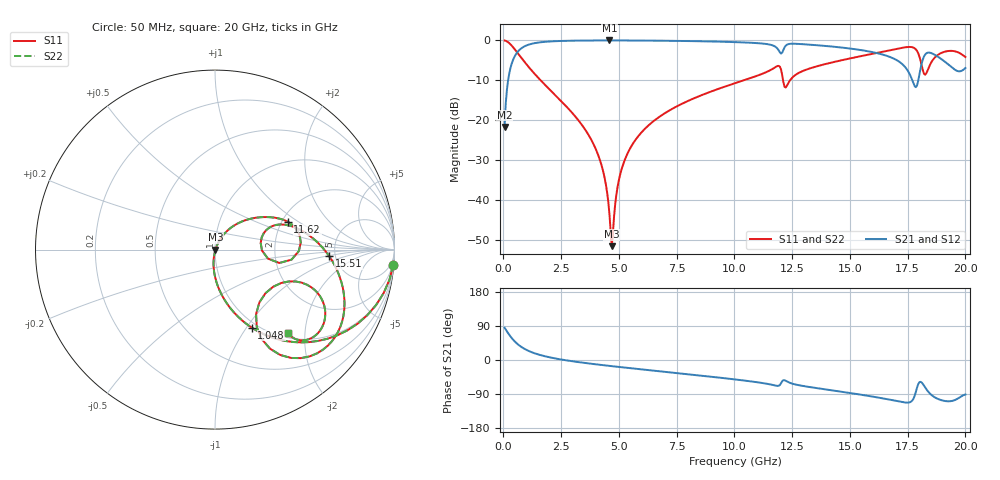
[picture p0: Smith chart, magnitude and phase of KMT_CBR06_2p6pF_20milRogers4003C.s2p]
! Data measured by Modelithics Inc. support@modelithics.com 813-866-6335
! KEMET CBR0603 2.6pF, Pad Width= 0.851mm, Pad Length= 0.64mm, Pad Gap= 0.62mm, 20mil Rogers 4003C substrate Data, January 2022
# hz S ma R 50
! 2 Port Network Data from SP1.SP block
! freq  magS11  angS11  magS21  angS21  magS12  angS12  magS22  angS22
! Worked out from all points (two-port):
!   401 points, 50 MHz to 20 GHz, reference 50 ohm
!   highest |S21| = -0.02 dB at 4.589 GHz (marker M1); lowest = -21.7 dB at 50 MHz (marker M2)
!   |S21| within 3 dB of the highest: 594.2 MHz to 11.97 GHz (11.38 GHz wide, 181 % of centre); 12.07 GHz to 16.04 GHz (3.97 GHz wide, 28.2 % of centre)
!   lowest |S11| = -51.5 dB at 4.688 GHz (marker M3), VSWR 1.01, Z = 50.2 - j0.0955 ohm
!   |S11| at or under -10 dB: 1.61 GHz to 10.4 GHz (8.794 GHz wide, 146 % of centre); 12.11 GHz to 12.41 GHz (302.9 MHz wide, 2.47 % of centre)
!   |S22| runs from -51.5 to 0.0 dB; largest |S21 - S12| = 0
!   S11 on the Smith chart (normalised r, x): 50 MHz: 1, -23; 1.048 GHz: 0.94, -1.06; 11.62 GHz: 2.15, +0.82; 15.51 GHz: 4.45, -0.56; 20 GHz: 1.09, -1.64
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5e7  0.9966 -4.9  0.08253 85.1  0.08253 85.1  0.9966 -4.9
3.99125e8  0.8321 -35.0  0.5537 54.9  0.5537 54.9  0.8321 -35.0
1.0475e9  0.4812 -64.7  0.8753 25.1  0.8753 25.1  0.4812 -64.7
3.391625e9  0.08784 -95.3  0.9938 -6.7  0.9938 -6.7  0.08784 -95.3
4.2395e9  0.02781 -97.9  0.997 -13.1  0.997 -13.1  0.02781 -97.9
4.588625e9  0.006676 -82.5  0.9972 -15.6  0.9972 -15.6  0.006676 -82.5
4.688375e9  0.002656 -21.0  0.9972 -16.2  0.9972 -16.2  0.002656 -21.0
4.987625e9  0.01726 62.6  0.9969 -18.2  0.9969 -18.2  0.01726 62.6
5.33675e9  0.03652 65.0  0.9963 -20.6  0.9963 -20.6  0.03652 65.0
6.73325e9  0.1095 58.7  0.9904 -29.5  0.9904 -29.5  0.1095 58.7
1.0025e10  0.2909 37.7  0.951 -51.2  0.951 -51.2  0.2909 37.7
1.1621e10  0.4341 20.9  0.8721 -65.3  0.8721 -65.3  0.4341 20.9
1.192025e10  0.4797 4.9  0.7465 -67.9  0.7465 -67.9  0.4797 4.9
1.22195e10  0.2572 8.3  0.8566 -54.8  0.8566 -54.8  0.2572 8.3
1.336662e10  0.455 16.2  0.8785 -72.4  0.8785 -72.4  0.455 16.2
1.551125e10  0.6376 -3.3  0.7533 -91.9  0.7533 -91.9  0.6376 -3.3
1.670825e10  0.7491 -17.5  0.6236 -104.5  0.6236 -104.5  0.7491 -17.5
1.78055e10  0.7948 -48.5  0.267 -94.3  0.267 -94.3  0.7948 -48.5
1.815462e10  0.4263 -57.5  0.5742 -62.9  0.5742 -62.9  0.4263 -57.5
1.8404e10  0.4486 -23.3  0.7033 -84.6  0.7033 -84.6  0.4486 -23.3
1.890275e10  0.6834 -27.1  0.5989 -104.9  0.5989 -104.9  0.6834 -27.1
2e10  0.6184 -48.7  0.451 -91.0  0.451 -91.0  0.6184 -48.7
